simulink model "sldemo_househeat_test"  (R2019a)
settings: Solver=VariableStepAuto  StartTime=0.0  StopTime=48  FixedStep=1  RelTol=1e-3  AbsTol=1e-6
model workspace (MATLAB code in the model file):
  other statements: sldemo_househeat_data
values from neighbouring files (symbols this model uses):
  c = 1005.4    [sldemo_househeat_data.m]
  cost = 0.09/3.6e6    (= 2.5e-08)    [sldemo_househeat_data.m]
  M = (lenHouse*widHouse*htHouse+tan(pitRoof)*widHouse*lenHouse)*densAir    [sldemo_househeat_data.m]
  Mdot = 3600    [sldemo_househeat_data.m]
  Req = RWall*RWindow/(RWall + RWindow)    [sldemo_househeat_data.m]
  THeater = 50    [sldemo_househeat_data.m]
  TinIC = 20    [sldemo_househeat_data.m]
libraries: simulink_extras x3

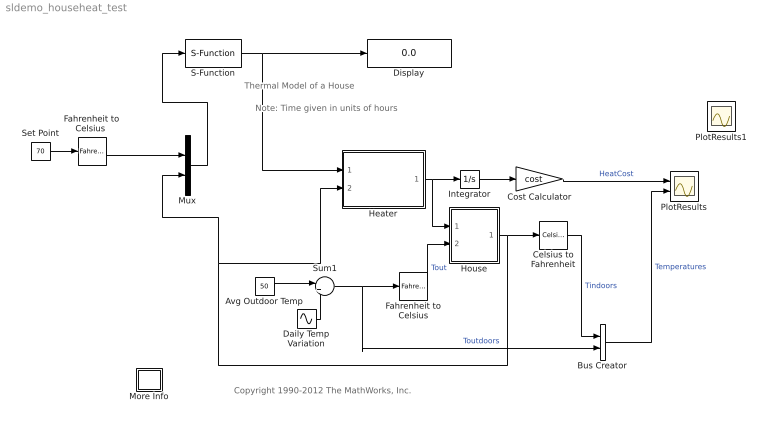
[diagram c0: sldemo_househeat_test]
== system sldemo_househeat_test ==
  note: Thermal Model of a House
  note: Copyright 1990-2012 The MathWorks, Inc.
  note: Note: Time given in units of hours
  Avg Outdoor Temp : Constant  Value=50
  Bus Creator : BusCreator  Inputs=2
  Celsius to Fahrenheit : simulink_extras/Transformations/Celsius to Fahrenheit
  Cost Calculator : Gain  Gain=cost
  Daily Temp Variation : Sin  Amplitude=15  Frequency=2*pi/24  SampleTime=0
  Display : Display
  Fahrenheit to Celsius : simulink_extras/Transformations/Fahrenheit to Celsius
  "Fahrenheit to Celsius " : simulink_extras/Transformations/Fahrenheit to Celsius
  Heater : Subsystem
  House : Subsystem
  Integrator : Integrator
  More Info : Subsystem
  Mux : Mux  Inputs=2
  PlotResults : Scope  NumInputPorts=2
  PlotResults1 : Scope  NumInputPorts=2
  S-Function : S-Function  FunctionName=modbusCom1  SFunctionDeploymentMode=off  EnableBusSupport=off
  Set Point : Constant  Value=70
  Sum1 : Sum  Inputs=|++
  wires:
  Integrator/1 -> Cost Calculator/1
  House/1(Room Temp Troom) -> Celsius to Fahrenheit/1, Mux/2, Heater/2(Troom)
  Daily Temp Variation/1 -> Sum1/2
  Sum1/1 -> Fahrenheit to Celsius/1, Bus Creator/2  "Toutdoors"
  Avg Outdoor Temp/1 -> Sum1/1
  Celsius to Fahrenheit/1 -> Bus Creator/1  "Tindoors"
  Fahrenheit to Celsius/1 -> House/2(Outdoor Temp Tout)  "Tout"
  Heater/1(HeatFlow) -> Integrator/1, House/1(Heater QDot In)
  Bus Creator/1 -> PlotResults/2  "Temperatures"
  Cost Calculator/1 -> PlotResults/1  "HeatCost"
  "Fahrenheit to Celsius "/1 -> Mux/1
  Set Point/1 -> "Fahrenheit to Celsius "/1
  S-Function/1 -> Heater/1(On/Off), Display/1
  Mux/1 -> S-Function/1

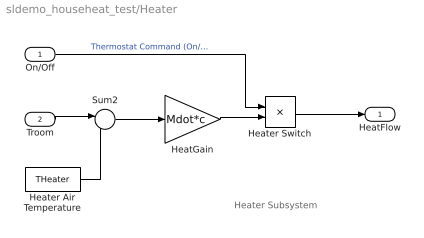
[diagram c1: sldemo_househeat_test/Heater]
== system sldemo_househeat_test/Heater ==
  note: Heater Subsystem
  On/Off : Inport
  Troom : Inport  Port=2
  HeatGain : Gain  Gain=Mdot*c
  Heater Air Temperature : Constant  Value=THeater
  Heater Switch : Product
  Sum2 : Sum  Inputs=|-+
  HeatFlow : Outport
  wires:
  Heater Air Temperature/1 -> Sum2/2
  Troom/1 -> Sum2/1
  Sum2/1 -> HeatGain/1
  On/Off/1 -> Heater Switch/1  "Thermostat Command (On/Off)"
  HeatGain/1 -> Heater Switch/2
  Heater Switch/1 -> HeatFlow/1

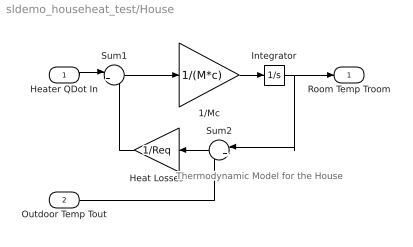
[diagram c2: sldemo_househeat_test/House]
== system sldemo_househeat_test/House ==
  note: Thermodynamic Model for the House
  Heater QDot In : Inport
  Outdoor Temp Tout : Inport  Port=2
  1/Mc : Gain  Gain=1/(M*c)
  Heat Losses : Gain  Gain=1/Req
  Integrator : Integrator  InitialCondition=TinIC
  Sum1 : Sum  Inputs=|+-
  Sum2 : Sum  Inputs=|+-
  Room Temp Troom : Outport  InitialOutput=0
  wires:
  Outdoor Temp Tout/1 -> Sum2/2
  Heater QDot In/1 -> Sum1/1
  Sum1/1 -> 1/Mc/1
  Sum2/1 -> Heat Losses/1
  Heat Losses/1 -> Sum1/2
  1/Mc/1 -> Integrator/1
  Integrator/1 -> Sum2/1, Room Temp Troom/1

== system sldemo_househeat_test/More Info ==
